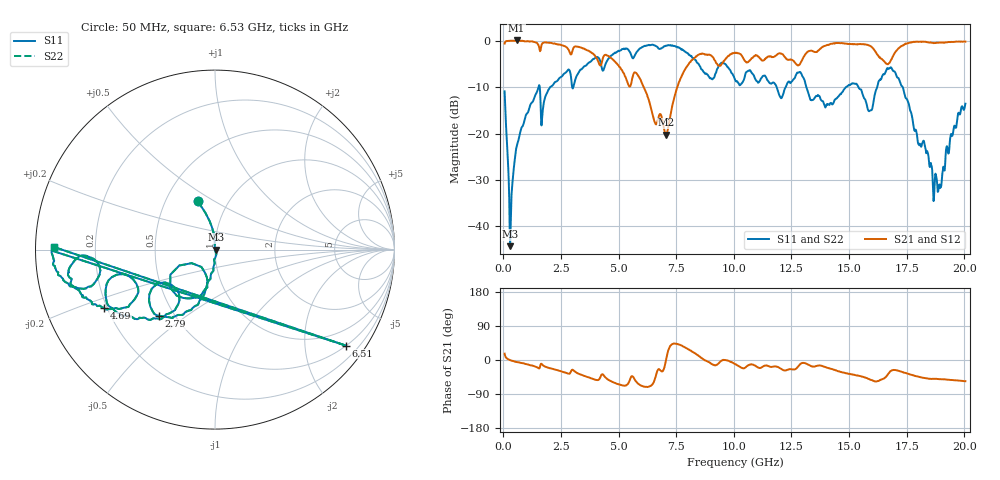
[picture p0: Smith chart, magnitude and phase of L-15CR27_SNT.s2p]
#	mhz	s	ma	r	50
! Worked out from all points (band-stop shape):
!   1001 points, 50 MHz to 20.05 GHz, reference 50 ohm
!   highest |S21| = 0.10 dB at 570 MHz (marker M1); lowest = -20.2 dB at 7.05 GHz (marker M2)
!   |S21| within 3 dB of the highest: 13.1 GHz to 16.22 GHz (3.12 GHz wide, 21.3 % of centre); 16.95 GHz to end of sweep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
!   lowest |S11| = -44.3 dB at 290 MHz (marker M3), VSWR 1.01, Z = 50.6 - j0.0406 ohm
!   |S11| at or under -10 dB: start of sweep to 1.52 GHz; 13.15 GHz to 14.86 GHz (1.71 GHz wide, 12.2 % of centre); 17.33 GHz to end of sweep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
!   |S22| runs from -44.3 to -0.8 dB; largest |S21 - S12| = 0
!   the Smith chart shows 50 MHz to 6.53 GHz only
!   S11 on the Smith chart (normalised r, x): 50 MHz: 0.72, +0.42; 2.79 GHz: 0.41, -0.40; 4.69 GHz: 0.19, -0.24; 6.51 GHz: 0.51, -2.97; 6.53 GHz: 0.05, +0.01
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50  0.286 109.6  0.937 16.8  0.937 16.8  0.286 109.6
290  0.00613 -3.8  1.004 -0.3  1.004 -0.3  0.00613 -3.8
570  0.07221 -92.0  1.012 -5.4  1.012 -5.4  0.07221 -92.0
1470  0.2888 -112.3  0.9414 -19.5  0.9414 -19.5  0.2888 -112.3
1710  0.1815 -103.5  0.9504 -13.7  0.9504 -13.7  0.1815 -103.5
2790  0.4826 -130.1  0.8242 -35.7  0.8242 -35.7  0.4826 -130.1
3390  0.4946 -129.1  0.8425 -39.2  0.8425 -39.2  0.4946 -129.1
4690  0.6989 -152.1  0.6498 -56.7  0.6498 -56.7  0.6989 -152.1
6510  0.9036 -36.3  0.1485 -60.1  0.1485 -60.1  0.9036 -36.3
6530  0.8971 179.1  0.1416 -57.7  0.1416 -57.7  0.8971 179.1
6730  0.8265 175.2  0.1487 -24.3  0.1487 -24.3  0.8265 175.2
7050  0.8888 170.4  0.09734 -1.5  0.09734 -1.5  0.8888 170.4
8130  0.6856 126.3  0.5983 24.8  0.5983 24.8  0.6856 126.3
10050  0.3823 115.9  0.7483 -10.7  0.7483 -10.7  0.3823 115.9
12850  0.4586 152.1  0.5538 -12.9  0.5538 -12.9  0.4586 152.1
13390  0.2298 136.9  0.7821 -16.9  0.7821 -16.9  0.2298 136.9
15230  0.346 68.5  0.9263 -39.1  0.9263 -39.1  0.346 68.5
15890  0.176 107.6  0.8898 -51.1  0.8898 -51.1  0.176 107.6
16730  0.5014 122.1  0.575 -34.4  0.575 -34.4  0.5014 122.1
17530  0.2308 65.3  0.9426 -35.7  0.9426 -35.7  0.2308 65.3
18750  0.03707 -88.9  0.9496 -49.7  0.9496 -49.7  0.03707 -88.9
20050  0.2105 -160.5  0.9823 -56.0  0.9823 -56.0  0.2105 -160.5
